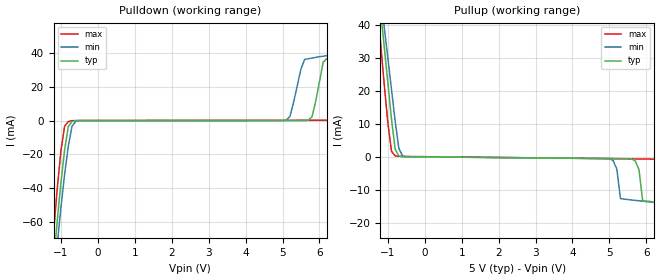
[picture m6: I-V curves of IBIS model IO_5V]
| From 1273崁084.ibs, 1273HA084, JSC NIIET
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[Model]   IO_5V
Model_type I/O
Polarity   Non-Inverting
Vinl =   0.80V
Vinh =   2.10V
C_comp   1.984800pF   1.899400pF   2.077500pF
[Temperature Range]   25   -60   85
[Voltage Range]   5.00V   4.50V   5.50V
[Pullup Reference]   5.00V   4.50V   5.50V
[Pulldown Reference]   0.00V   0.00V   0.00V
[POWER Clamp Reference]   5.00V   4.50V   5.50V
[GND Clamp Reference]   0.00V   0.00V   0.00V
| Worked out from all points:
|   slope of the pullup table from 0 to 0.75 V, typ, clamps not added: 9.99 kohm
[Pullup]
| Voltage   I(typ)   I(min)   I(max)
-5.5V     781.6mA    688mA      936mA
-1.2V     44.75mA    49.8mA     35.13mA
-1.1V     33.76mA    39.66mA    22.4mA
-900mV    11.44mA    20.51mA    1.693mA
-700mV    258.9uA    2.526mA    165.1uA
5V        -496.7uA   -527.6uA   -535uA
5.3V      -528uA     -12.65mA   -572.1uA
5.6V      -593.6uA   -13.05mA   -609.5uA
5.9V      -13.24mA   -13.42mA   -647.2uA
6.2V      -13.63mA   -13.79mA   -725uA
6.5V      -14mA      -14.17mA   -13.6mA
11V       -20.7mA    -23.13mA   -21.95mA
[Pulldown]
| Voltage   I(typ)   I(min)   I(max)
-5.5V     -1.524A    -1.383A    -1.74A
-1.2V     -84.36mA   -96.66mA   -66.72mA
-1.1V     -59.65mA   -73.56mA   -40.53mA
-900mV    -17.44mA   -31.85mA   -3.355mA
-800mV    -3.591mA   -15.23mA   -623.4uA
-600mV    -49.04uA   -442.4uA   -24.41uA
5.1V      7.504uA    257uA      132.2uA
5.7V      210.2uA    36.65mA    146.6uA
6.1V      34.64mA    38.14mA    156.6uA
6.3V      37.16mA    38.87mA    275.4uA
6.7V      38.55mA    40.41mA    32.71mA
11V       53.41mA    55.43mA    53.08mA
[Ramp]
| variable   typ   min   max
dV/dt_r   1.1447/1.0797n   0.8477/2.2066n   1.3962/0.5592n
dV/dt_f   1.1301/1.6088n   0.6820/2.6083n   1.4669/0.8614n
R_load = 1500ohms
